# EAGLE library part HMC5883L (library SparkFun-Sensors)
Honewell HMC5883L 3 Axis Digital Compass IC a 3-axis digital magnetometer designed for low-field magnetic sensing. The sensor has a full-scale range of ±8 Guass and a resolution of up to 5 milli-Gauss. Supplied voltage should be between 2.16 and 3.6VDC. Communication with the HMC5883L is simple and all done through an I2C interface. All registers and operating modes are well described in the datasheet below. Datasheet SparkFun Products Magnetometer Digital Triple Axis - HMC5883L (COM-10494) SparkFun Triple Axis Magnetometer Breakout - HMC5883L (SEN-10530) 9 Degrees of Freedom - Razor IMU (SEN-10736) SparkFun 9 Degrees of Freedom - Sensor Stick (SEN-10724)
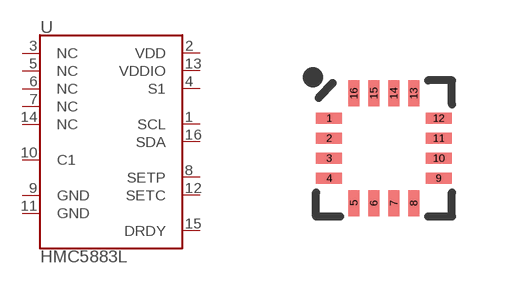
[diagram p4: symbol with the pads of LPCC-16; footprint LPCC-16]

Designator prefix U

## HMC5883L (PROD_ID: IC-10284; SF_ID: COM-10494)  [LPCC-16]
1  SCL
2  VDD
3  NC
4  S1
5  NC
6  NC
7  NC
8  SETP
9  GND
10  C1
11  GND
12  SETC
13  VDDIO
14  NC
15  DRDY
16  SDA

## Footprint LPCC-16 (pad centres in mm)
16-Pin LCC (3 x 3 x 0.9 mm) Datasheet Specifications: Pin Count: 16 Area: 3.0 x 3.0 x 0.9 mm Pitch: 0.5 mm Devices Using: HMC5883L
smd 0.65 x 0.28: 1 -1.37,0.75; 2 -1.37,0.25; 3 -1.37,-0.25; 4 -1.37,-0.75; 9 1.37,-0.75; 10 1.37,-0.25; 11 1.37,0.25; 12 1.37,0.75
smd 0.28 x 0.65: 5 -0.75,-1.37; 6 -0.25,-1.37; 7 0.25,-1.37; 8 0.75,-1.37; 13 0.75,1.37; 14 0.25,1.37; 15 -0.25,1.37; 16 -0.75,1.37

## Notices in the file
Licensing: Creative Commons ShareAlike 4.0 International - https://creativecommons.org/licenses/by-sa/4.0
